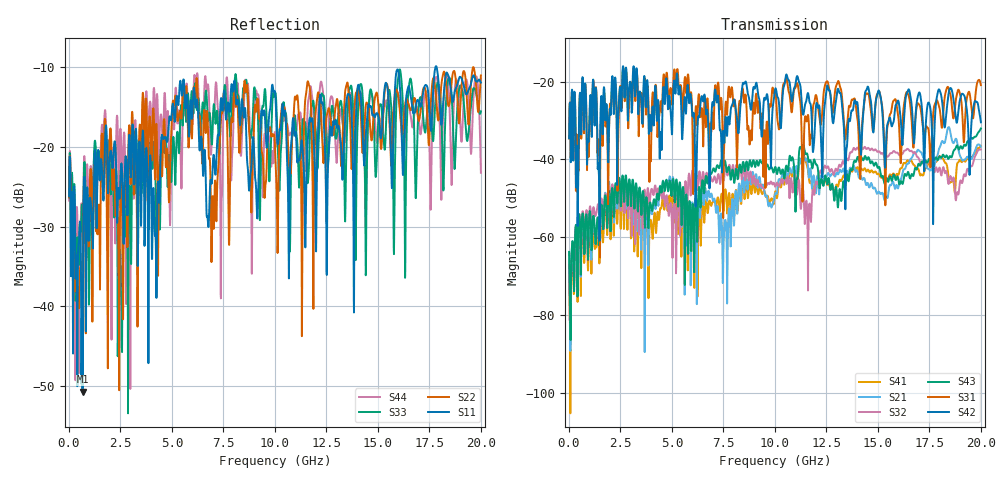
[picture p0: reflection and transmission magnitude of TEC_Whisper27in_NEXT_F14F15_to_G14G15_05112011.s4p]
! Tyco Electronics
! F14F15-G14G15_NEXT
!! PART DESCRIPTION: Whisper 27in Megtron 6 VLP-HVLP-VLP Channel Model, bulkhead 2.4mm test pts
!! MODEL DESCRIPTION: System 4-port S-parameter
!! MODEL STATUS: Measured
!! MODEL GEOMETRY: Channel Model
!! MODEL FREQUENCY RANGE: DC to 20.000 GHz in 10.000 MHz frequency steps
!! MODEL EDGE RATE LIMITATION: 25.00 ps (Using conservative 0.5/Fmax rule of thumb)
!! TIME-DOMAIN TRANSFORM CAUTIONS:
!! 1.) Do not simulate transient edge rates faster than the number listed above.  Edge rates faster than this number
!!  contain significant spectral content at frequencies above the model's highest frequency.
!! 2.) Even when simulating edge rates that are slower than the number listed above, be aware that the best time
!!  resolution possible with a direct iFFT is (1 / 2Fmax).  As a result, time resolution is typically not adequate
!!  for most time-domain simulations unless tricks such as windowing are used to minimize leakage and aliasing.
!! 3.) Because the model has a uniform frequency step, a direct iFFT will result in an impulse that that has a time
!!  length given by either (1 / Fstep) or (1 / 2Fstep), depending on the transform being used.  Care has been taken
!!  in selecting the frequency step to ensure a settled impulse response for the model.  Therefore, convolution with
!!  the model's impulse response should present no issues.  However, if directly concatenating s-parameter models
!!  in the frequency domain a user must either interpolate necessary interim frequencies or complete impulse response
!!  zero-padding.  Impulse response zero-padding is more difficult, but more accurate.
!! PORT DEFINITIONS:
!! Port  1  ----->  Side A  F14  G14  Side A  <-----  Port  2
!! Port  3  ----->  Side A  F15  G15  Side A  <-----  Port  4
! Point-to-Point link (differential)  !
! Connectors:  !
!  1: STRADA Whisper  !
! Materials:  !
!  Backplane: Megtron-6 HVLP  !
!  Daughtercard: Megtron-6 VLP  !
! Stack-up:  !
!  Backplane: 20 layers, 200mil thick  !
!  Daughtercard: 14 layers, 110mil thick  !
! Trace Length:  !
!  Backplane: 17in  !
!  Daightercards: 5in  !
! Trace Width:  !
!  Backplane: 8-13-8 mils  !
!  Daughtercards: 6-9-6 mils  !
! Geometry:  !
!  Backplane: Stripline  !
!  Daughtercards: Stripline  !
! Freq. Range: 0 GHz - 20 GHz  !
! Note1: non-mixed-mode s-parameters  !
! Note2: channel includes 2.4mm test points  !
! Created Wed May 11 14:58:56 2011
! 4 Port Network Data from SP1.SP block
! freq  magS11  angS11  magS12  angS12  magS13  angS13  magS14  angS14
!  magS21  angS21  magS22  angS22  magS23  angS23  magS24  angS24
!  magS31  angS31  magS32  angS32  magS33  angS33  magS34  angS34
!  magS41  angS41  magS42  angS42  magS43  angS43  magS44  angS44
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# hz S ma R 50
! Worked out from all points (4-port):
!   2000 points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, 10 MHz to 20 GHz, reference 50 ohm
!   strongest paths, dB at 10 MHz, 5.01 GHz, 10.01 GHz, 15.01 GHz, 20 GHz:
!     S42: -34.5, -33.2, -22.0, -22.5, -30.4
!     S31: -34.6, -25.4, -22.5, -22.8, -20.9
!     S43: -63.7, -47.3, -42.0, -42.1, -32.0
!     S32: -67.0, -59.6, -47.0, -38.0, -37.4
!     S21: -63.8, -45.8, -48.9, -48.4, -36.7
!     S41: -67.6, -49.7, -48.4, -43.7, -36.5
!   lowest |S11| = -50.7 dB at 660 MHz (marker M1), VSWR 1.01, Z = 50.1 - j0.275 ohm
!   |S11| at or under -10 dB: start of sweep to 17.79 GHz; 17.85 GHz to end of sweep
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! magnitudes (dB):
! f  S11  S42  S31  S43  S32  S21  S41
! 10 MHz  -26.2  -34.5  -34.6  -63.7  -67.0  -63.8  -67.6
! 660 MHz  -50.7  -18.8  -19.3  -53.9  -53.4  -54.2  -57.4
! 5.48 GHz  -13.5  -32.5  -23.1  -56.2  -47.8  -55.4  -59.1
! 6.75 GHz  -29.4  -29.5  -25.7  -45.7  -45.7  -48.6  -53.5
! 10.6 GHz  -22.3  -18.8  -20.1  -42.4  -45.4  -44.4  -45.2
! 15.38 GHz  -11.9  -38.7  -45.8  -45.3  -39.2  -49.5  -45.3
! 20 GHz  -11.9  -30.4  -20.9  -32.0  -37.4  -36.7  -36.5
